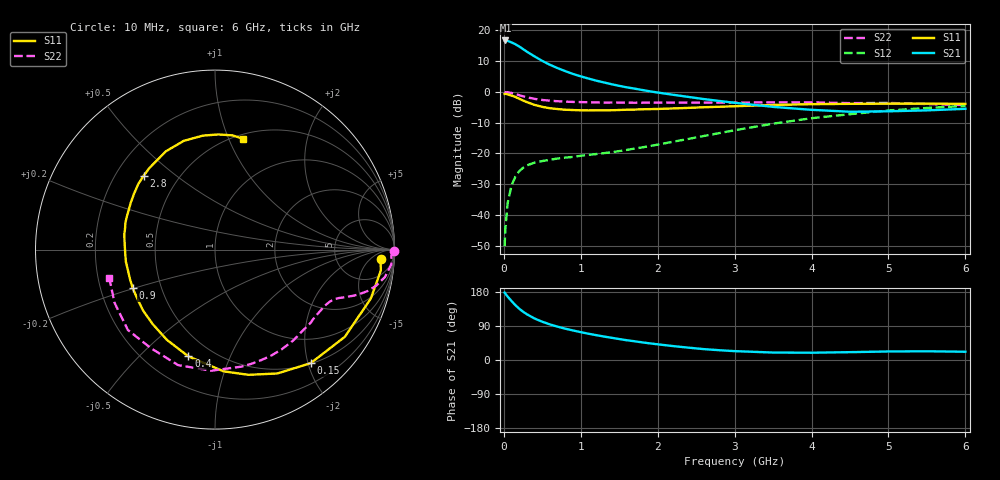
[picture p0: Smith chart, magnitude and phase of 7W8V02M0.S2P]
! Infineon Technologies  Discrete & RF Semiconductors
! BFS17W
! Si NPN RF Bipolar Junction Transistor in SOT323
! VCE = 8 V  IC = 2 mA
! Common Emitter S-Parameters:  August  1999
# GHz  S  MA  R  50
!  f  S11  S21  S12  S22
! GHz  MAG  ANG  MAG  ANG  MAG  ANG  MAG  ANG
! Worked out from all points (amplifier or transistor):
!   36 points, 10 MHz to 6 GHz, reference 50 ohm
!   highest |S21| = 16.7 dB at 20 MHz (marker M1)
!   |S21| within 3 dB of that: start of sweep to 261.2 MHz
!   unconditionally stable (mu >= 1): 855.8 MHz to 2.743 GHz; 4.383 GHz to end of sweep
!   at 250 MHz: K = 0.35, MSG = 19.3 dB, |S12| = -24.7 dB
!   at 1.4 GHz: K = 1.26, MAG = 8.0 dB, |S12| = -19.6 dB
!   at 6 GHz: K = 1.08, MAG = -2.2 dB, |S12| = -4.6 dB
!   S11 on the Smith chart (normalised r, x): 10 MHz: 16, -12; 150 MHz: 0.51, -2.05; 400 MHz: 0.37, -0.71; 900 MHz: 0.34, -0.20; 2.8 GHz: 0.32, +0.39; 6 GHz: 0.54, +1.13
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0.01  0.9241 -3.4  6.836 178.0  0.0031 82.3  0.9999 -0.5
0.02  0.9313 -7.2  6.845 175.0  0.006 88.0  0.9837 -1.8
0.05  0.9098 -17.5  6.728 167.2  0.0157 82.4  0.9861 -4.8
0.1  0.8714 -33.9  6.368 155.7  0.0301 72.2  0.9589 -9.2
0.15  0.8273 -49.9  5.944 144.6  0.0418 63.4  0.9202 -12.6
0.2  0.7726 -63.3  5.454 135.4  0.0513 59.3  0.8827 -15.1
0.25  0.7223 -75.0  4.953 127.4  0.0581 53.2  0.8448 -17.0
0.3  0.6802 -85.9  4.491 120.7  0.0637 50.1  0.8162 -18.3
0.4  0.6131 -104.0  3.757 109.4  0.0709 45.1  0.7688 -20.2
0.5  0.5697 -118.1  3.183 101.0  0.075 42.8  0.738 -21.5
0.6  0.5413 -129.8  2.748 93.8  0.0788 42.5  0.7181 -22.8
0.7  0.5253 -139.7  2.426 87.9  0.0825 43.1  0.7039 -24.2
0.9  0.5061 -155.1  1.952 77.9  0.0875 44.7  0.6855 -27.4
1.1  0.4986 -167.4  1.645 69.3  0.0943 48.1  0.6767 -31.1
1.3  0.5007 -177.5  1.423 61.9  0.1008 51.8  0.6703 -35.3
1.6  0.5124 170.2  1.183 52.1  0.1139 57.5  0.6659 -41.7
2.2  0.5375 150.8  0.896 36.7  0.1546 66.9  0.6683 -56.3
2.8  0.5719 134.1  0.711 25.8  0.2134 70.1  0.6679 -72.3
3.5  0.6121 116.6  0.57 19.7  0.3039 67.7  0.6751 -91.8
4.5  0.6386 96.1  0.475 20.7  0.4332 56.0  0.6552 -123.0
5.5  0.6438 81.4  0.5 23.0  0.5468 42.4  0.6333 -152.1
6  0.6371 76.0  0.53 21.8  0.5908 35.8  0.6097 -165.1
